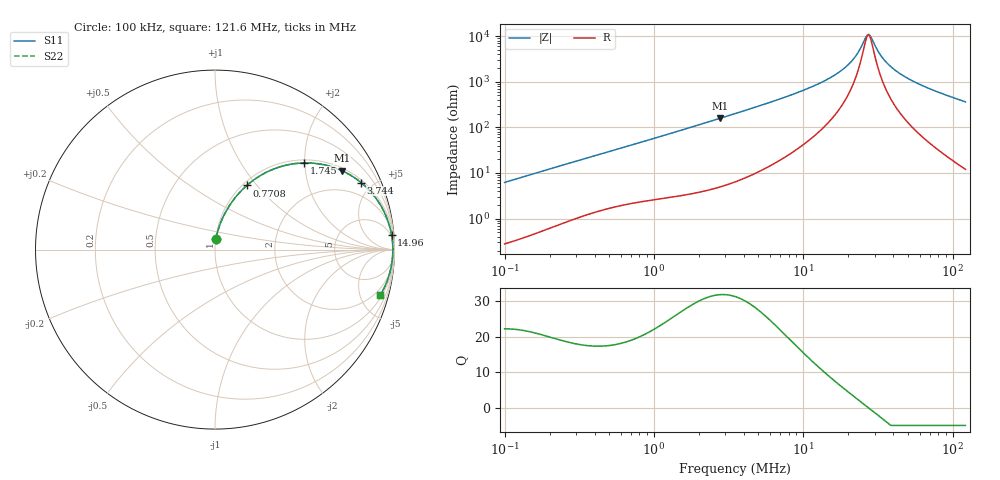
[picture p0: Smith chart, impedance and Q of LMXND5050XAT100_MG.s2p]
! LMXND5050XAT100_MG  S-PARAMETER MODEL  ( General Type )
! Model Generated by TAIYO YUDEN Corporation (https://www.yuden.co.jp/en/)
! Version 1.0
! TAIYO YUDEN Control No. 191023NI43SB-FBB
! Copyright(c) 2019 TAIYO YUDEN CO.,LTD. All Rights Reserved.
! Product Description (link to TY-COMPAS)
! https://ds.yuden.co.jp/TYCOMPAS/or/detail?pn=LMXND5050XAT100MMG&u=M
! Products Name : Inductors
! Characteristics :
!  Inductance : 10 uH , SRF(min) : 20 MHz , DC Resistance(max) : 0.091 Ohm
!  Rated Current : Saturation :2100 mA , Temp Rise : 1700 mA (40 degC)
!  Case Size : 4.9 x 4.9 / 0.193 x 0.193 [mm/inch] , Thickness : 3.1 / 0.122 [mm/inch]
!  (Conditions: Temperature = 25 degC , DC Bias Current/Voltage = 0A / 0V)
! External Node Assignments :
!  1  o---GGG---o  2
! GND o---------o GND
! Frequency Range : 0.1MHz  -  121.638923MHz  [ 402 STEP ]
# MHz S RI R 50
! Freq[MHz].  S11 Real  S11 Imag  S21 Real  S21 Imag  S12 Real  S12 Imag  S22 Real  S22 Imag
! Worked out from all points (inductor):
!   401 points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, 100 kHz to 121.6 MHz, reference 50 ohm
!   read as one part in series: L = 9.83 uH near 103.6 kHz
!   highest Q = 31.9 at 2.769 MHz (marker M1), where L = 9.06 uH
!   self-resonance near 26.88 MHz
!   S11 on the Smith chart (normalised r, x): 100 kHz: 1.01, +0.12; 770.8 kHz: 1.05, +0.89; 1.745 MHz: 1.07, +1.98; 3.744 MHz: 1.14, +4.30; 14.96 MHz: 4, +24; 121.6 MHz: 1.24, -7.24
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0.1  0.00659 0.0615  0.9934 -0.0615  0.9934 -0.0615  0.00659 0.0615
0.328662  0.0472 0.1857  0.9528 -0.1857  0.9528 -0.1857  0.0472 0.1857
0.77083  0.1776 0.3576  0.8224 -0.3576  0.8224 -0.3576  0.1776 0.3576
1.080188  0.2845 0.4299  0.7155 -0.4299  0.7155 -0.4299  0.2845 0.4299
1.744784  0.4958 0.4829  0.5042 -0.4829  0.5042 -0.4829  0.4958 0.4829
2.768671  0.7074 0.4396  0.2926 -0.4396  0.2926 -0.4396  0.7074 0.4396
3.550168  0.7978 0.386  0.2022 -0.386  0.2022 -0.386  0.7978 0.386
3.744441  0.8142 0.3731  0.1858 -0.3731  0.1858 -0.3731  0.8142 0.3731
6.156616  0.9212 0.2495  0.0788 -0.2495  0.0788 -0.2495  0.9212 0.2495
11.46267  0.9748 0.1233  0.0252 -0.1233  0.0252 -0.1233  0.9748 0.1233
14.96153  0.984 0.081  0.016 -0.081  0.016 -0.081  0.984 0.081
18.18929  0.9879 0.0532  0.0121 -0.0532  0.0121 -0.0532  0.9879 0.0532
20.96607  0.9896 0.0341  0.0104 -0.0341  0.0104 -0.0341  0.9896 0.0341
23.32347  0.9904 0.0202  0.00957 -0.0202  0.00957 -0.0202  0.9904 0.0202
26.41082  0.9909 0.00418  0.00914 -0.00418  0.00914 -0.00418  0.9909 0.00418
27.36575  0.9909 -0.000363  0.00912 0.000363  0.00912 0.000363  0.9909 -0.000363
28.3552  0.9909 -0.00491  0.00913 0.00491  0.00913 0.00491  0.9909 -0.00491
33.26954  0.9903 -0.0255  0.00974 0.0255  0.00974 0.0255  0.9903 -0.0255
37.67347  0.9892 -0.0419  0.0108 0.0419  0.0108 0.0419  0.9892 -0.0419
45.80101  0.9861 -0.0689  0.0139 0.0689  0.0139 0.0689  0.9861 -0.0689
58.729  0.9793 -0.1067  0.0207 0.1067  0.0207 0.1067  0.9793 -0.1067
121.6389  0.9221 -0.252  0.0779 0.252  0.0779 0.252  0.9221 -0.252
